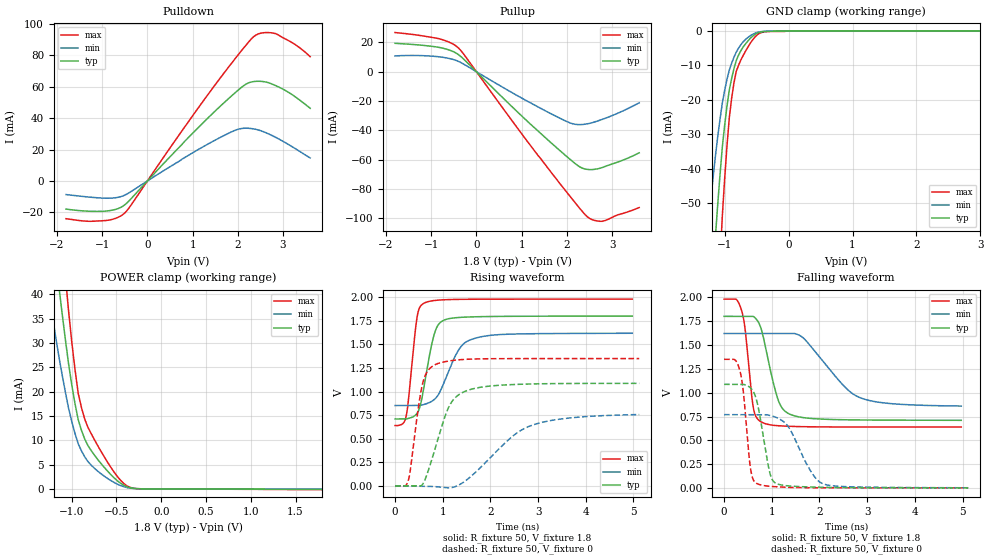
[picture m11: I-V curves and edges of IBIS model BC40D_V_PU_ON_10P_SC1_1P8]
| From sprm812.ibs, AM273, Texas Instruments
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|   Model Cell BC40D_V_PU_ON_10P_SC1_1P8
|BC40D_V_PU_ON_10P_SC1_1P8
[Model]   BC40D_V_PU_ON_10P_SC1_1P8
Model_type   I/O
Polarity   Non-Inverting
Enable   Active-Low
Vinl =  0.63
Vinh =  1.17
Cref =  15pF
Rref =  100.0000M
Vref =  0V
Vmeas =  0.9
C_comp   2.290246p   2.205796p   2.292736p
|[Input load] weak_pu_on
|[Output drive] slow
|[supplytol] 10
|[temp] ind
[Model Spec]
Vinl   0.63   0.567   0.693
Vinh   1.17   1.053   1.287
[Temperature Range]   25   125   -40
[Voltage Range]   1.8   1.62   1.98
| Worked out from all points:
|   slope of the pulldown table from 0 to 0.27 V, typ, clamps not added: 32.2 ohm
|   slope of the pullup table from 0 to 0.27 V, typ, clamps not added: 32.6 ohm
|   GND clamp passes 1 mA (typ) near -0.52 V on its own axis
|   POWER clamp passes 1 mA (typ) near -0.44 V on its own axis
|   rising waveform, R_fixture 50, V_fixture 1.8: 20-80 % time 245ps typ, 416ps min, 160ps max; typ from 0.711 V to 1.8 V
|   rising waveform, R_fixture 50, V_fixture 0: 20-80 % time 428ps typ, 996ps min, 229ps max; typ from 0.002 V to 1.09 V
|   falling waveform, R_fixture 50, V_fixture 1.8: 20-80 % time 308ps typ, 788ps min, 165ps max; typ from 1.8 V to 0.71 V
|   falling waveform, R_fixture 50, V_fixture 0: 20-80 % time 226ps typ, 462ps min, 150ps max; typ from 1.09 V to 0.002 V
| Nom Voltages:
|   VDD=1.1001, VDDS=1.8, VDDS18=1.8, ESD_BIASFET=0, VSS=0, VSSS=0
| Min Voltages:
|   VDD=0.99, VDDS=1.62, VDDS18=1.62, ESD_BIASFET=0, VSS=0, VSSS=0
| Max Voltages:
|   VDD=1.21, VDDS=1.98, VDDS18=1.98, ESD_BIASFET=0, VSS=0, VSSS=0
[POWER_clamp]
|   voltage   I(typ)   I(min)   I(max)
-1.8V     158.8mA    112.5mA    219.8mA
-1.255V   59.97mA    40.01mA    84.9mA
-1.145V   41.92mA    27.42mA    59.75mA
-1.109V   36.32mA    23.63mA    51.82mA
-1.073V   30.96mA    20.05mA    44.15mA
-1.036V   25.83mA    16.67mA    36.75mA
-963.6mV  17.54mA    11.39mA    24.55mA
-890.9mV  12.01mA    7.801mA    16.66mA
-818.2mV  8.875mA    5.6mA      12.63mA
-563.6mV  2.954mA    1.727mA    4.458mA
-272.7mV  55.97uA    39.41uA    57.82uA
1.8V      -99.94uA   -59.68uA   -146.8uA
[Pulldown]
|   voltage   I(typ)   I(min)   I(max)
-1.8V     -17.92mA   -8.674mA   -24.03mA
-927.3mV  -19.22mA   -10.99mA   -25.21mA
-654.5mV  -17.65mA   -10.46mA   -23.22mA
-490.9mV  -14.97mA   -8.904mA   -20.12mA
818.2mV   25.06mA    14.78mA    34.16mA
1.691V    49.7mA     28.87mA    68.59mA
2.127V    60.63mA    33.53mA    84.59mA
2.4V      63.43mA    32.84mA    92.9mA
2.618V    62.99mA    30.74mA    94.47mA
2.836V    60.69mA    27.76mA    93.76mA
3.273V    53.49mA    20.53mA    86.73mA
3.6V      46.26mA    14.64mA    79.12mA
[Pullup]
|   voltage   I(typ)   I(min)   I(max)
-1.8V     19.42mA    10.82mA    26.76mA
-818.2mV  16.58mA    10.15mA    22.47mA
-545.5mV  14.19mA    8.648mA    19.37mA
-381.8mV  11.34mA    6.842mA    15.75mA
1.036V    -31.26mA   -18.6mA    -43.9mA
1.909V    -55.59mA   -32.73mA   -78.89mA
2.182V    -62.71mA   -35.92mA   -89.46mA
2.345V    -65.94mA   -36.05mA   -95.62mA
2.455V    -66.75mA   -35.58mA   -99.18mA
2.618V    -66.67mA   -34.29mA   -101.7mA
2.782V    -65.47mA   -32.56mA   -102.2mA
3.6V      -55.4mA    -21.22mA   -92.82mA
[GND_clamp]
|   voltage   I(typ)   I(min)   I(max)
-1.8V     -270.2mA   -170.2mA   -430.1mA
-1.255V   -91.68mA   -55.92mA   -148.5mA
-1.145V   -59.94mA   -36.46mA   -97.15mA
-1.109V   -50.51mA   -30.84mA   -81.62mA
-1.073V   -41.77mA   -25.67mA   -67.14mA
-1.036V   -33.71mA   -20.94mA   -53.69mA
-927.3mV  -17.15mA   -11.38mA   -25.2mA
-854.5mV  -10.96mA   -7.657mA   -15.09mA
-781.8mV  -7.031mA   -4.995mA   -9.958mA
-563.6mV  -1.569mA   -1.036mA   -2.651mA
-18.18mV  0A         0A         0A
3.6V      0A         0A         0A
[Ramp]
| variable   typ   min   max
dV/dt_f 0.66095897/0.31060812n 0.46741276/0.81020272n 0.80998719/0.16631685n
dV/dt_r 0.65862638/0.43190449n 0.47366209/1.0494131n 0.81474121/0.23003732n
R_load = 50
[Rising Waveform]
R_fixture = 50
V_fixture = 1.8
V_fixture_min = 1.62
V_fixture_max = 1.98
|   time   V(typ)   V(min)   V(max)
0s        710.6mV    852.8mV    640.5mV
228.8ps   710.6mV    852.8mV    730.4mV
277.8ps   716.3mV    852.8mV    897.5mV
460.2ps   769.7mV    852.8mV    1.785V
608.1ps   1.054V     864.3mV    1.937V
831.2ps   1.624V     920.4mV    1.966V
1.058ns   1.764V     1.135V     1.974V
1.377ns   1.787V     1.474V     1.978V
1.755ns   1.794V     1.576V     1.979V
4.974ns   1.8V       1.618V     1.98V
[Rising Waveform]
R_fixture = 50
V_fixture = 0
V_fixture_min = 0
V_fixture_max = 0
|   time   V(typ)   V(min)   V(max)
0s        2.031mV    0V         2.114mV
277.7ps   2.031mV    0V         58.72mV
569.5ps   13.14mV    -2.708mV   1.069V
672.4ps   127.3mV    -2.903mV   1.21V
825.7ps   372.3mV    -5.554mV   1.282V
1.153ns   863.3mV    -18.47mV   1.326V
1.54ns    1.017V     80.39mV    1.344V
2.425ns   1.074V     510.5mV    1.35V
2.844ns   1.081V     638.7mV    1.35V
5.12ns    1.088V     757.1mV    1.35V
[Falling Waveform]
R_fixture = 50
V_fixture = 1.8
V_fixture_min = 1.62
V_fixture_max = 1.98
|   time   V(typ)   V(min)   V(max)
0s        1.8V       1.62V      1.981V
368.4ps   1.8V       1.62V      1.86V
440.1ps   1.8V       1.62V      1.67V
613.3ps   1.799V     1.62V      843.1mV
788ps     1.653V     1.62V      690.9mV
1.123ns   939.8mV    1.62V      653.8mV
1.375ns   775.1mV    1.62V      647mV
1.663ns   738.3mV    1.573V     643.3mV
2.826ns   713.9mV    953mV      639.9mV
4.974ns   710.1mV    859.9mV    639.7mV
[Falling Waveform]
R_fixture = 50
V_fixture = 0
V_fixture_min = 0
V_fixture_max = 0
|   time   V(typ)   V(min)   V(max)
0s        1.087V     769.6mV    1.35V
327.6ps   1.087V     769.6mV    1.238V
402.9ps   1.087V     769.6mV    1.014V
550.7ps   1.052V     769.6mV    218.7mV
679.6ps   925.5mV    769.6mV    49.18mV
952.7ps   172.9mV    762.4mV    18.54mV
1.106ns   45.55mV    737.5mV    13.56mV
1.354ns   22.29mV    637.9mV    7.313mV
2.087ns   7.614mV    42.5mV     3.032mV
5.12ns    2.077mV    3.234mV    2.564mV
